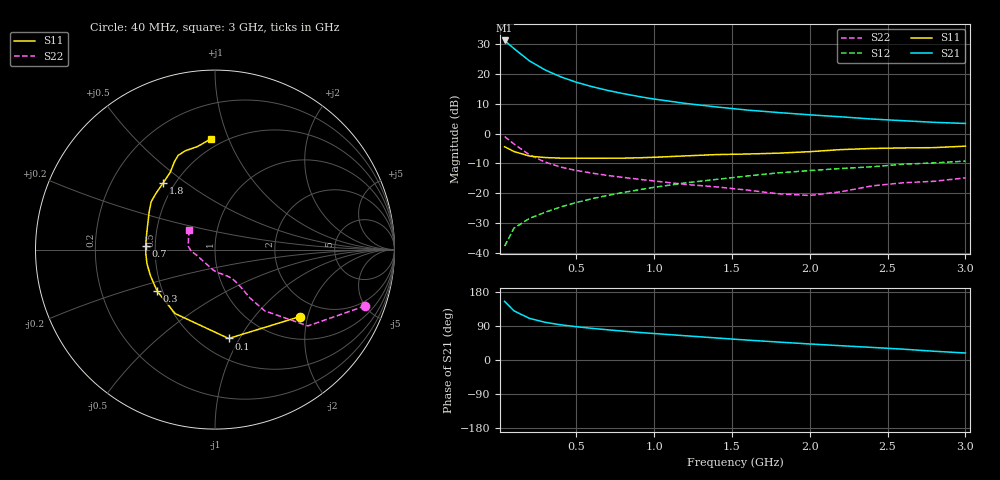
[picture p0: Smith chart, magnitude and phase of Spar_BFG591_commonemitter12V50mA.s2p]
! Filename:  BFG591E.S2P  Version:  4.0
! NXP part #: BFG591  Date: Jun 1994
! Bias condition: Vce=12V; Ic=50mA
#  MHz  S  MA  R  50
! Freq  S11  S21  S12  S22  !GUM [dB]
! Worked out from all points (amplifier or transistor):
!   21 points, 40 MHz to 3 GHz, reference 50 ohm
!   highest |S21| = 31.2 dB at 40 MHz (marker M1)
!   |S21| within 3 dB of that: start of sweep to 106.7 MHz
!   unconditionally stable (mu >= 1): 650.9 MHz to 2.189 GHz
!   at 300 MHz: K = 0.82, MSG = 23.9 dB, |S12| = -26.4 dB
!   at 1 GHz: K = 1.05, MAG = 13.5 dB, |S12| = -18.0 dB
!   at 3 GHz: K = 0.95, MSG = 6.3 dB, |S12| = -9.2 dB
!   S11 on the Smith chart (normalised r, x): 40 MHz: 1.52, -1.79; 100 MHz: 0.68, -0.90; 300 MHz: 0.47, -0.26; 700 MHz: 0.44, +0.02; 1.8 GHz: 0.43, +0.41; 3 GHz: 0.43, +0.86
40  0.602 -38.4  36.34 154.7  0.013 74.4  0.893 -20.6
100  0.501 -81.3  26.55 129.7  0.026 62.7  0.67 -39.4
200  0.42 -121.9  16.5 109.8  0.038 59.5  0.44 -50.9
300  0.397 -144.1  11.66 99.5  0.048 61.3  0.333 -54.1
400  0.388 -158.0  8.95 92.9  0.059 63.3  0.275 -55.0
500  0.387 -168.1  7.258 87.9  0.07 65.3  0.241 -55.9
600  0.386 -176.0  6.129 83.6  0.081 65.9  0.218 -57.0
700  0.387 177.3  5.304 79.8  0.092 66.5  0.199 -58.3
800  0.388 170.9  4.683 76.2  0.103 66.6  0.185 -59.9
900  0.393 164.7  4.193 72.9  0.114 66.7  0.172 -62.4
1000  0.401 159.1  3.793 69.9  0.126 66.5  0.161 -65.6
1200  0.423 150.1  3.208 64.0  0.149 65.2  0.141 -74.4
1400  0.445 143.0  2.797 58.2  0.171 63.5  0.128 -84.8
1600  0.455 136.0  2.477 52.5  0.195 62.5  0.113 -96.2
1800  0.47 128.0  2.251 47.3  0.22 59.5  0.098 -110.9
2000  0.498 120.0  2.063 42.3  0.24 57.9  0.092 -137.5
2200  0.539 114.8  1.911 37.7  0.26 55.6  0.106 -162.6
2400  0.564 111.3  1.754 33.2  0.278 54.7  0.133 -176.2
2600  0.575 106.6  1.644 28.6  0.307 51.1  0.15 172.8
2800  0.582 99.8  1.544 23.1  0.323 47.2  0.159 158.7
3000  0.616 92.3  1.479 18.5  0.346 45.7  0.181 142.2
